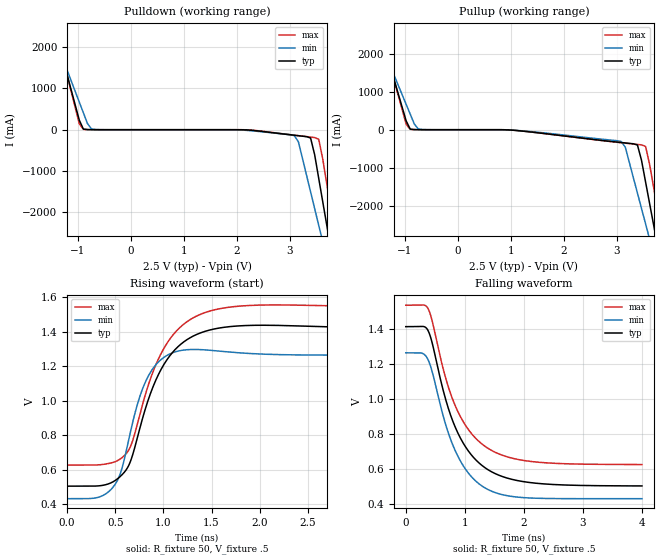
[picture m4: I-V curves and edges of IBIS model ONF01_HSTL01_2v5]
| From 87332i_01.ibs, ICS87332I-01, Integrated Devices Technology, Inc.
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[Model] ONF01_HSTL01_2v5
Model_type  Output_ECL
Polarity   Non-Inverting
Vmeas = .89
Rref = 50
Cref = 0
Vref = .5
|Variable  typ   min   max
C_comp   2p   1.5p   2.5p
[Voltage Range]   2.5   2.375   2.625
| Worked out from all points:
|   rising waveform, R_fixture 50, V_fixture .5: 20-80 % time 350ps typ, 240ps min, 362ps max; typ from 0.504 V to 1.42 V
|   falling waveform, R_fixture 50, V_fixture .5: 20-80 % time 591ps typ, 523ps min, 591ps max; typ from 1.41 V to 0.504 V
| Open source, no load
|  Voltage   I(typ)   I(min)   I(max)
[Pullup]
-2.5V     7.585A     5.853A     7.966A
-1.582V   3.168A     2.738A     3.268A
-1.505V   2.8A       2.478A     2.877A
-892.9mV  15.1mA     409.7mA    8.262mA
-739.8mV  1.385mA    17.35mA    1.003mA
3.087V    -338.1mA   -312.6mA   -343.9mA
3.393V    -404.5mA   -1.675A    -388.5mA
3.469V    -807.4mA   -2.079A    -400mA
3.546V    -1.379A    -2.483A    -441.2mA
3.699V    -2.523A    -3.292A    -1.528A
3.852V    -3.666A    -4.1A      -2.744A
5V        -12.24A    -10.16A    -11.86A
[Pulldown]
-2.5V     7.585A     5.853A     7.966A
-1.505V   2.8A       2.478A     2.877A
-1.429V   2.433A     2.219A     2.485A
-892.9mV  15.1mA     409.7mA    8.262mA
-663.3mV  413.9uA    3.764mA    253.1uA
3.087V    -134.5mA   -144.5mA   -132.9mA
3.393V    -201.7mA   -1.506A    -178.4mA
3.469V    -604.8mA   -1.91A     -190.2mA
3.546V    -1.177A    -2.315A    -231.7mA
3.699V    -2.321A    -3.123A    -1.319A
3.852V    -3.464A    -3.931A    -2.535A
5V        -12.04A    -9.99A     -11.65A
[Ramp]
|   typ   min   max
dV/dt_r   0.747/0.607n   0.692/0.422n   0.743/0.611n
dV/dt_f   0.728/0.954n   0.666/0.82n   0.729/0.951n
R_load =   50.0000
[Rising Waveform]
R_fixture = 50
V_fixture = .5   | VCC_typ - 2V
V_fixture_max = 0.625   | VCC_max - 2V
V_fixture_min = 0.375   | VCC_min - 2V
C_fixture = 0.0p
| Time   typ   min   max
0s        503.5mV    430.9mV    625.7mV
426.4ps   516.2mV    469mV      634.6mV
537.1ps   552.3mV    553.7mV    655.9mV
615ps     599.4mV    709mV      693.2mV
725.7ps   775.8mV    969.5mV    854.9mV
824.1ps   972.5mV    1.121V     1.055V
1.099ns   1.282V     1.278V     1.38V
1.365ns   1.389V     1.296V     1.496V
1.755ns   1.433V     1.279V     1.547V
3.997ns   1.415V     1.264V     1.538V
[Falling Waveform]
R_fixture = 50
V_fixture = .5   | VCC_typ - 2V
V_fixture_max = 0.625   | VCC_max - 2V
V_fixture_min = 0.375   | VCC_min - 2V
C_fixture = 0.0p
| Time   typ   min   max
0s        1.413V     1.264V     1.536V
270.6ps   1.415V     1.262V     1.537V
373.1ps   1.394V     1.228V     1.519V
446.9ps   1.321V     1.157V     1.446V
668.3ps   1.006V     861.8mV    1.129V
832.3ps   843.5mV    708.9mV    965.8mV
1.074ns   696.6mV    571.2mV    819.3mV
1.365ns   602.2mV    488mV      724.4mV
2.148ns   521.3mV    434.3mV    642.4mV
3.997ns   503.9mV    431mV      626mV
